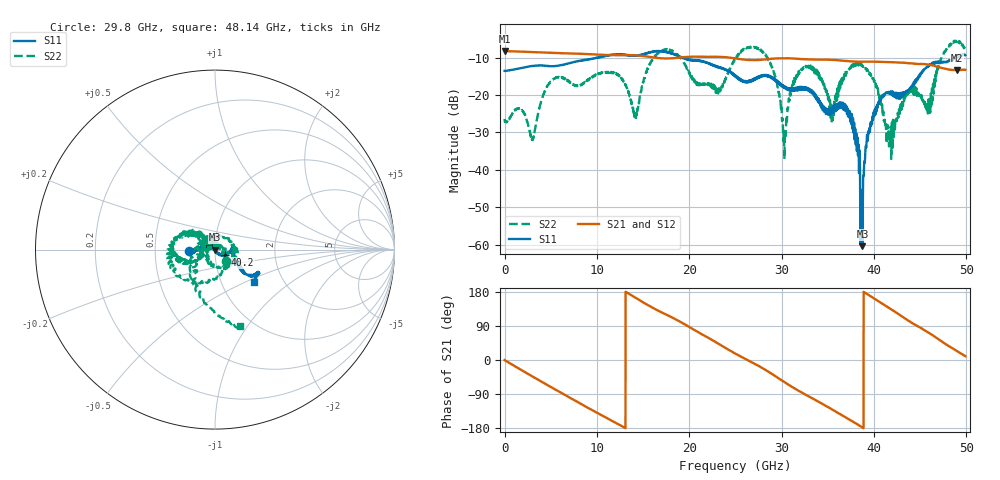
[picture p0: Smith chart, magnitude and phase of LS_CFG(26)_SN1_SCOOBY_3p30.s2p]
!Keysight Technologies,N5245B,MY58422026,A.13.80.08
!Date: Thursday, March 19, 2020 23:34:53
!Correction: S11(Full 2 Port(1,2))
!S21(Full 2 Port(1,2))
!S12(Full 2 Port(1,2))
!S22(Full 2 Port(1,2))
!S2P File: Measurements: S11, S21, S12, S22:
# Hz S DB R 50.0
!freq dBS11 angS11 dBS21 angS21 dBS12 angS12 dBS22 angS22
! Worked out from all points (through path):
!   4991 points, 10 MHz to 49.91 GHz, reference 50 ohm
!   highest |S21| = -8.28 dB at 10 MHz (marker M1); lowest = -13.4 dB at 49.01 GHz (marker M2)
!   group delay of S21, straight-line fit = 39.1 ps
!   lowest |S11| = -60.4 dB at 38.76 GHz (marker M3), VSWR 1.00, Z = 50.1 - j0.0457 ohm
!   |S11| at or under -10 dB: start of sweep to 10.05 GHz; 10.09 GHz to 10.15 GHz (56.99 MHz wide, 0.563 % of centre); 19.22 GHz to 48.76 GHz (29.53 GHz wide, 86.9 % of centre)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
!   |S22| runs from -37.1 to -5.4 dB; largest |S21 - S12| = 0.0038
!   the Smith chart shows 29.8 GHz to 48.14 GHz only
!   S11 on the Smith chart (normalised r, x): 29.8 GHz: 0.75, -0.01; 40.2 GHz: 1.12, -0.07; 48.14 GHz: 1.43, -0.56
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1e7  -13.57 -1.1  -8.28 -0.2  -8.26 -0.3  -26.39 1.0
3.02e9  -12.28 -34.1  -8.54 -43.3  -8.53 -43.3  -31.73 -73.4
5.04e9  -12.32 -53.8  -8.76 -71.6  -8.76 -71.6  -16.28 -106.8
8.33e9  -10.84 -79.7  -9.01 -116.6  -9.00 -116.6  -17.23 -96.5
1.209e10  -9.12 -106.5  -9.38 -166.4  -9.37 -166.4  -14.29 -87.5
1.419e10  -9.52 -123.3  -9.41 164.4  -9.41 164.4  -25.80 -132.8
1.665e10  -8.30 -134.9  -10.13 130.1  -10.12 130.2  -8.79 -164.7
2.312e10  -12.64 -169.2  -9.81 43.6  -9.81 43.8  -19.59 -154.3
2.496e10  -14.79 -172.4  -10.20 17.4  -10.18 17.5  -10.54 -170.4
2.786e10  -14.81 -171.4  -10.61 -20.5  -10.60 -20.3  -8.20 -97.2
2.98e10  -16.74 -177.0  -10.20 -50.2  -10.21 -50.1  -20.92 -46.6
3.036e10  -18.15 -176.8  -10.19 -59.0  -10.19 -58.8  -31.16 49.5
3.328e10  -18.94 177.9  -10.51 -100.6  -10.51 -100.3  -12.61 -170.1
3.553e10  -24.29 137.8  -10.62 -131.3  -10.55 -131.0  -26.80 170.0
3.74e10  -24.97 136.8  -11.00 -157.9  -10.93 -158.0  -12.83 162.1
3.876e10  -60.37 -28.4  -11.12 -178.1  -11.09 -178.4  -12.12 -141.6
4.02e10  -23.81 -27.0  -11.10 159.7  -11.08 159.4  -17.38 -74.1
4.16e10  -19.24 7.6  -11.21 138.0  -11.24 137.8  -30.01 98.7
4.59e10  -12.19 -37.3  -11.89 72.4  -11.91 72.5  -21.38 118.9
4.814e10  -10.92 -39.4  -13.19 36.5  -13.20 36.5  -6.96 -72.3
4.901e10  -9.59 -47.7  -13.36 23.4  -13.38 23.4  -5.44 -43.0
4.991e10  -9.36 -43.7  -13.27 10.1  -13.30 10.0  -8.02 -14.9
